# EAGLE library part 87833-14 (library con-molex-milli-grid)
HEADER
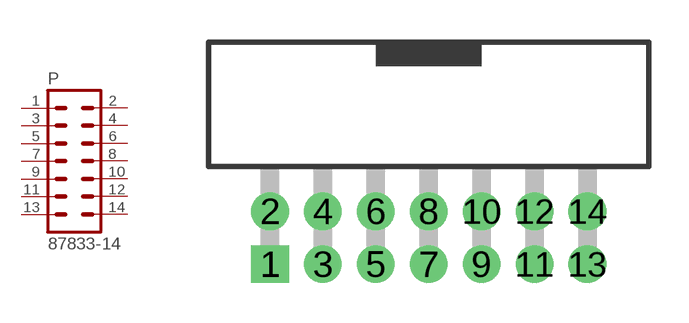
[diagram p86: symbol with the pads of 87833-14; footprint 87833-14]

Designator prefix P

## 87833-14  [87833-14]
1  1  pas
2  2  pas
3  3  pas
4  4  pas
5  5  pas
6  6  pas
7  7  pas
8  8  pas
9  9  pas
10  10  pas
11  11  pas
12  12  pas
13  13  pas
14  14  pas

## Footprint 87833-14 (pad centres in mm)
HEADER Dual Row, Shrouded, Right Angle
drill 0.914 square: 1 -6,-1
drill 0.914: 2 -6,1; 3 -4,-1; 4 -4,1; 5 -2,-1; 6 -2,1; 7 0,-1; 8 0,1; 9 2,-1; 10 2,1; 11 4,-1; 12 4,1; 13 6,-1; 14 6,1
